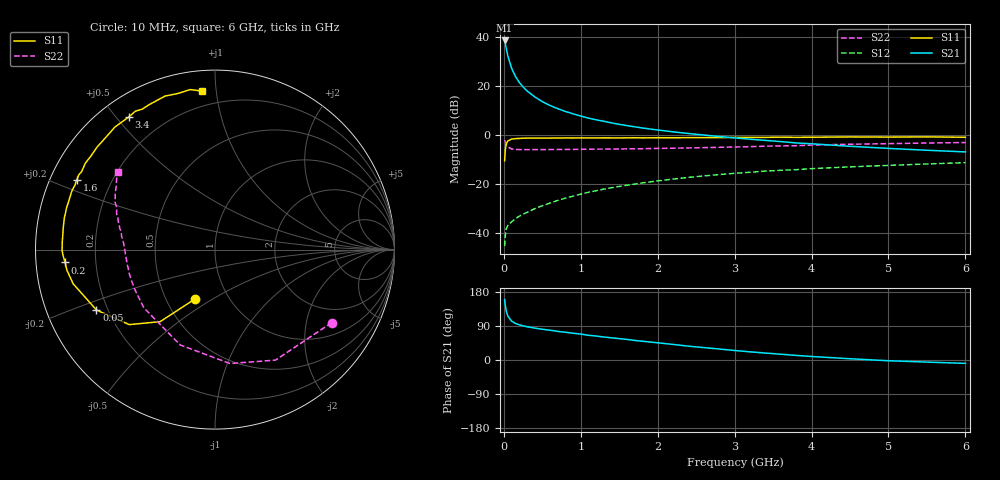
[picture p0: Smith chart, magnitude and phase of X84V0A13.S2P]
! SIEMENS Small Signal Semiconductors
! BFP136W
! Si NPN RF Bipolar Junction Transistor in SOT343
! VCE = 4 V  IC = 130 mA
! Common Emitter S-Parameters:  September  1994
# GHz  S  MA  R  50
!  f  S11  S21  S12  S22
! GHz  MAG  ANG  MAG  ANG  MAG  ANG  MAG  ANG
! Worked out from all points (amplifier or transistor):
!   40 points, 10 MHz to 6 GHz, reference 50 ohm
!   highest |S21| = 38.5 dB at 10 MHz (marker M1)
!   |S21| within 3 dB of that: start of sweep to 29.84 MHz
!   unconditionally stable (mu >= 1): 490.8 MHz to 2.951 GHz; 3.792795 GHz to 3.810149 GHz
!   at 200 MHz: K = 0.72, MSG = 27.3 dB, |S12| = -33.3 dB
!   at 1.5 GHz: K = 1.11, MAG = 10.6 dB, |S12| = -21.1 dB
!   at 6 GHz: K = 0.97, MSG = 2.2 dB, |S12| = -11.4 dB
!   S11 on the Smith chart (normalised r, x): 10 MHz: 0.70, -0.42; 50 MHz: 0.16, -0.23; 200 MHz: 0.09, -0.04; 1.6 GHz: 0.08, +0.24; 3.4 GHz: 0.08, +0.54; 6 GHz: 0.11, +0.92
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0.01  0.2943 -111.7  83.89 159.4  0.0053 68.2  0.7673 -32.0
0.02  0.5047 -127.3  71.08 142.4  0.0089 54.8  0.702 -61.3
0.03  0.6346 -138.8  59.21 130.5  0.0117 49.5  0.6402 -82.5
0.05  0.7412 -153.0  41.76 116.7  0.0139 38.7  0.5657 -110.0
0.1  0.8125 -166.4  22.89 102.8  0.0166 39.2  0.5121 -140.7
0.15  0.8327 -172.0  15.55 96.6  0.0192 41.7  0.4991 -153.1
0.2  0.838 -175.1  11.68 92.9  0.0217 43.2  0.4963 -159.8
0.25  0.8473 -177.8  9.419 90.1  0.0239 46.3  0.4958 -164.1
0.3  0.8521 -179.7  7.876 88.0  0.0259 48.7  0.4947 -166.9
0.4  0.8521 176.8  5.932 84.2  0.0308 53.1  0.4962 -170.9
0.5  0.8519 174.3  4.728 81.1  0.0354 55.9  0.4968 -173.5
0.6  0.8538 172.2  3.943 78.6  0.0402 57.7  0.4976 -175.3
0.7  0.8561 169.5  3.403 75.5  0.0455 59.6  0.4994 -176.6
0.9  0.8575 166.2  2.663 70.6  0.0557 60.8  0.5012 -179.2
1.1  0.8582 162.0  2.178 65.3  0.0667 61.4  0.5049 179.2
1.6  0.8627 153.1  1.532 54.3  0.0928 59.5  0.5137 175.1
2.2  0.8658 142.9  1.143 41.1  0.1239 55.1  0.5284 170.5
3.2  0.8803 126.0  0.808 21.5  0.1711 45.6  0.5699 161.8
3.4  0.8812 123.0  0.765 18.3  0.1807 43.5  0.5828 160.1
4.5  0.8995 108.0  0.58 3.3  0.2203 33.4  0.6378 150.6
5.5  0.9023 98.8  0.481 -5.5  0.2525 25.5  0.6763 144.1
6  0.886 94.6  0.445 -8.9  0.2687 21.2  0.6913 141.2
